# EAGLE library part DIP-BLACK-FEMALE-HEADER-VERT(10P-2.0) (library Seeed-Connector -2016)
320030009
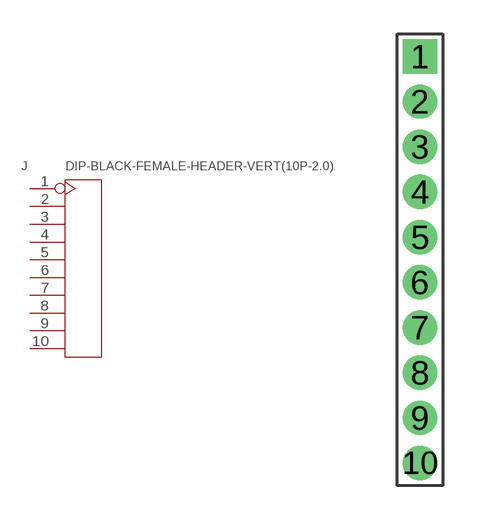
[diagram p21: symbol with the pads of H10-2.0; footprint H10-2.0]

Designator prefix J

## DIP-BLACK-FEMALE-HEADER-VERT(10P-2.0) (MPN: F243-1110A1BSUA1; VALUE: 10p-2.0)  [H10-2.0]
1  1
2  2
3  3
4  4
5  5
6  6
7  7
8  8
9  9
10  10

## Footprint H10-2.0 (pad centres in mm)
drill 0.813 pad 1.524 square: 1 0,9
drill 0.813 pad 1.524: 2 0,7; 3 0,5; 4 0,3; 5 0,1; 6 0,-1; 7 0,-3; 8 0,-5; 9 0,-7; 10 0,-9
